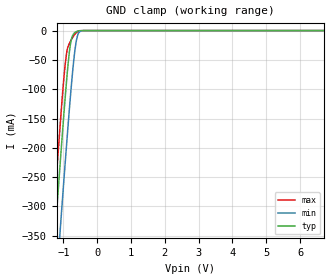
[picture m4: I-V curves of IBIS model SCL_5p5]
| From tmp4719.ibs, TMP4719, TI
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|   Model
[Model]   SCL_5p5
Model_type   Input
Vinl = .99
Vinh = 2.31
|   typ   min   max
C_comp   1.19pF   1.17pF   1.22pF
[Voltage Range]   5.5   5   6.1
[Temperature Range]   25   125   -40
[Power Clamp Reference]   5.5   5   6.1
[GND Clamp Reference]   0   0   0
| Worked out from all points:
|   GND clamp passes 1 mA (typ) near -0.58 V on its own axis
[GND Clamp]
|   Voltage   I(typ)   I(min)   I(max)
-4.7V     -3.272A    -3.37A     -3.22A
-1.344V   -429.2mA   -543.9mA   -362.8mA
-1.161V   -280.9mA   -395.7mA   -214.3mA
-1.076V   -214.1mA   -328.5mA   -148.3mA
-977.6mV  -138.8mA   -251.4mA   -77.66mA
-907.1mV  -88.44mA   -197.7mA   -40.08mA
-780.2mV  -20.37mA   -106.3mA   -17.55mA
-681.5mV  -4.681mA   -46.07mA   -8.082mA
-611mV    -1.702mA   -16.41mA   -3.377mA
-526.4mV  -285.9uA   -2.396mA   -515.8uA
-385.4mV  -3.102uA   -49.33uA   -1.758uA
9.4V      0A         0A         0A
